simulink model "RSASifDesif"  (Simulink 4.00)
settings: Solver=ode45  StartTime=0.0  StopTime=10.0  RelTol=1e-3

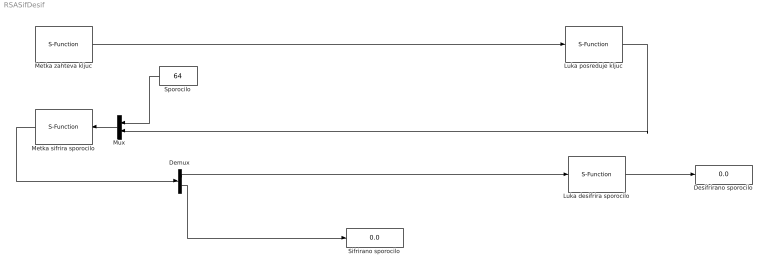
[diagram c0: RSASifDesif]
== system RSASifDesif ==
  Demux : Demux  Outputs=2  BusSelectionMode=off
  Desifrirano sporocilo : Display
  Luka desifrira sporocilo : S-Function  FunctionName=desifrirajSporocilo  Parameters=37,527  PortCounts=[]  SFunctionModules=''
  Luka posreduje kljuc : S-Function  FunctionName=posredujKljuc  Parameters=13,527  PortCounts=[]  SFunctionModules=''
  Metka sifrira sporocilo : S-Function  Orientation=left  FunctionName=sifrirajSporocilo  PortCounts=[]  SFunctionModules=''
  Metka zahteva kljuc : S-Function  FunctionName=pridobiKljuc  PortCounts=[]  SFunctionModules=''
  Mux : Mux  Orientation=left  Inputs=2
  Sifrirano sporocilo : Display
  Sporocilo : Constant  Orientation=left  Value=64
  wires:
  Luka desifrira sporocilo/1 -> Desifrirano sporocilo/1
  Metka zahteva kljuc/1 -> Luka posreduje kljuc/1
  Metka sifrira sporocilo/1 -> Demux/1
  Sporocilo/1 -> Mux/1
  Mux/1 -> Metka sifrira sporocilo/1
  Demux/1 -> Luka desifrira sporocilo/1
  Demux/2 -> Sifrirano sporocilo/1
  Luka posreduje kljuc/1 -> Mux/2
